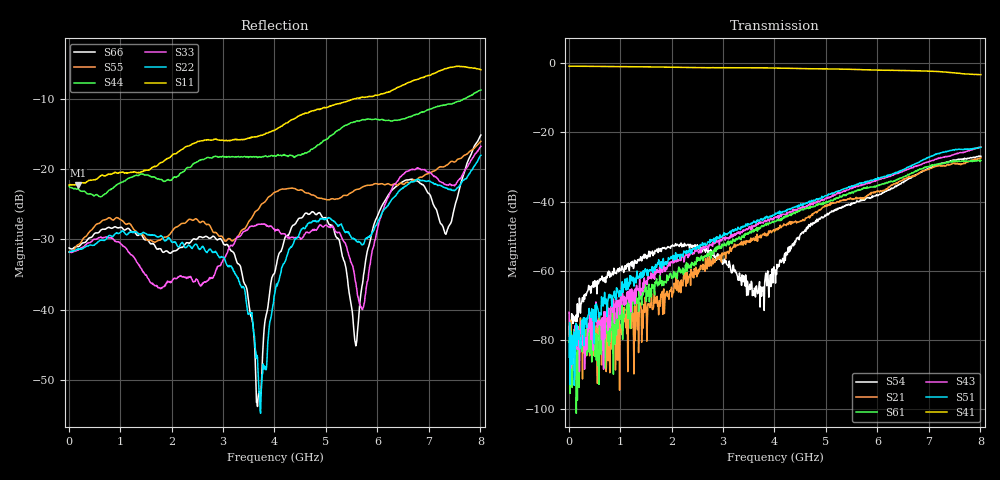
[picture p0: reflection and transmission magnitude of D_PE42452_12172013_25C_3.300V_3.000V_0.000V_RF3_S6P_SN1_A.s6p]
! Device ID: PE42422_06252012
! Dir: z:\David_A\42452\10_28_13_42452_omar_meas\25C\3p300000\RF3
! Serial: 1
! Insertion: A
! Temp: 25C
! VDD: 3.300
! Control_Hi: 3.000
! Control_Lo: 0.000
! Logic State: RF3
! Port 1: RFC
! Port 2: RF1
! Port 3: RF2
! Port 4: RF3
! Port 5: RF4
! Port 6: RF5
! ThroughPath:4-1
! V1 = 3.00
! V2 = 3.00
! V3 = 0.00
! V4 = 0.00
#  Hz  S  RI  R  50
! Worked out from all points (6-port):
!   801 points, 10 MHz to 8.01 GHz, reference 50 ohm
!   strongest paths, dB at 10 MHz, 2.01 GHz, 4.01 GHz, 6.01 GHz, 8.01 GHz:
!     S41: -0.8, -1.1, -1.4, -1.9, -3.2
!     S51: -85.0, -56.5, -43.5, -33.0, -24.3
!     S43: -72.0, -57.7, -44.6, -33.5, -24.2
!     S61: -80.4, -62.0, -45.8, -35.3, -28.1
!     S21: -80.8, -67.6, -48.1, -37.0, -27.3
!     S54: -76.1, -52.8, -60.0, -38.3, -26.9
!   lowest |S11| = -22.3 dB at 180 MHz (marker M1), VSWR 1.17, Z = 58.1 - j1.84 ohm
!   |S11| at or under -10 dB: start of sweep to 5.553 GHz; 5.57308 GHz to 5.582007 GHz (8.927 MHz wide, 0.16 % of centre)
